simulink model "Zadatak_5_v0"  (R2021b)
settings: Solver=VariableStepAuto  StartTime=0.0  StopTime=0.2  RelTol=1e-3
libraries: ee_lib x5, fl_lib x4, nesl_utility x3, spsSequenceAnalyzerLib x1

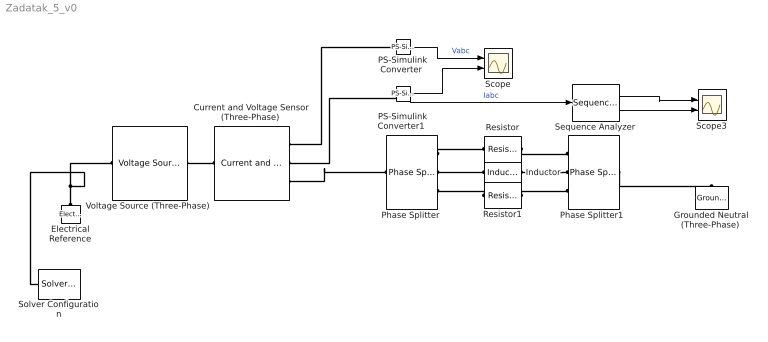
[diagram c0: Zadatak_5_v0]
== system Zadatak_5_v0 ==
  "Current and Voltage Sensor (Three-Phase) " : ee_lib/Sensors & Transducers/Current and Voltage Sensor (Three-Phase)  vMeasurementType=ee.enum.vmeasurement.lg  outputUnit=ee.enum.unit.si  SRated=100e6 V*A  VRated=24e3 V  I_specify=off  I_priority=None  I=[ 0 0 0 ] A  I_nominal_specify=off  I_nominal_unit=A  I_nominal_value=1  V_specify=off  V_priority=None  V=[ 0 0 0 ] V  V_nominal_specify=off  V_nominal_unit=V  V_nominal_value=1
  Electrical Reference : fl_lib/Electrical/Electrical Elements/Electrical Reference
  "Grounded Neutral (Three-Phase) " : ee_lib/Connectors & References/Grounded Neutral (Three-Phase)
  Inductor : fl_lib/Electrical/Electrical Elements/Inductor  l=1 H  r=0 Ohm  g=1e-9 1/Ohm  i_specify=off  i_priority=None  i=0 A  i_nominal_specify=off  i_nominal_unit=A  i_nominal_value=1  v_specify=off  v_priority=None  v=0 V  v_nominal_specify=off  v_nominal_unit=V  v_nominal_value=1  i_L_specify=off  i_L_priority=High  i_L=0 A  i_L_nominal_specify=off  i_L_nominal_unit=A  i_L_nominal_value=1
  "PS-Simulink Converter " : nesl_utility/PS-Simulink Converter  PhysicalDomain=network_engine_domain  SubClassName=ps_output  LeftPortType=input  RightPortType=output  PseudoPeriodic=off  Frequencies=[]  Unit=inherit  AffineConversion=off
  "PS-Simulink Converter1 " : nesl_utility/PS-Simulink Converter  PhysicalDomain=network_engine_domain  SubClassName=ps_output  LeftPortType=input  RightPortType=output  PseudoPeriodic=off  Frequencies=[]  Unit=inherit  AffineConversion=off
  "Phase Splitter " : ee_lib/Connectors & References/Phase Splitter
  "Phase Splitter1 " : ee_lib/Connectors & References/Phase Splitter
  Resistor : fl_lib/Electrical/Electrical Elements/Resistor  R=1000 Ohm  i_specify=off  i_priority=None  i=0 A  i_nominal_specify=off  i_nominal_unit=A  i_nominal_value=1  v_specify=off  v_priority=None  v=0 V  v_nominal_specify=off  v_nominal_unit=V  v_nominal_value=1
  Resistor1 : fl_lib/Electrical/Electrical Elements/Resistor  R=1000 Ohm  i_specify=off  i_priority=None  i=0 A  i_nominal_specify=off  i_nominal_unit=A  i_nominal_value=1  v_specify=off  v_priority=None  v=0 V  v_nominal_specify=off  v_nominal_unit=V  v_nominal_value=1
  Scope : Scope  NumInputPorts=2
  Scope3 : Scope  NumInputPorts=2
  "Sequence Analyzer " : spsSequenceAnalyzerLib/Sequence Analyzer  Freq=50  n=1  seq=Positive Negative Zero  InInit=[1, 0]  Ts=0
  Solver Configuration : nesl_utility/Solver Configuration  PhysicalDomain=network_engine_domain  SubClassName=solver  LeftPortType=input  RightPortType=generic  Tones=[]  Harmonics=[]  SimulateNoise=off  Profile=off  UseLocalSampling=off  EnableSwitchedLinearOptims=on  FrequencyDomain=off  UseCCode=off  RelTol=0.001  AbsTol=1e-06  MinStep=1e-09  ToWorkspace=off  RevertToSquareIcSolve=off  NumHomotopyIterations=100  PhasorMode=off  PhasorModeNumHarmonics=1  DoDC=on  ResidualTolerance=1e-09  UseLocalSolver=off  LocalSolverChoice=NE_BACKWARD_EULER_ADVANCER  LocalSolverSampleTime=0.001  DoFixedCost=off  MaxNonlinIter=3  MaxModeIter=2  ComputeImpulses=off  ImpulseIterations=2  LinearAlgebra=auto  EquationFormulation=NE_TIME_EF  DelaysMemoryBudget=1024  AutomaticFiltering=on  FilteringTimeConstant=0.001  PartitionStorageMethod=AS_NEEDED  PartitionMemoryBudget=1024  PartitionMethod=ROBUST
  "Voltage Source (Three-Phase) " : ee_lib/Sources/Voltage Source (Three-Phase)  vline_rms=380 V  shift=0 deg  freq=50 Hz  impedance_option=0  SShortCircuit=1e6 V*A  XR=15  R=0.01 Ohm  L=3.97e-4 H  harmonic_option=0  harmonic_orders=[5, 7, 11, 13]  harmonic_ratios=[.1, .1, .1, .1]  G_parasitic=0 1/Ohm  I_specify=off  I_priority=None  I=[ 0 0 0 ] A  I_nominal_specify=off  I_nominal_unit=A  I_nominal_value=1
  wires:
  "PS-Simulink Converter "/1 -> Scope/1  "Vabc"
  "PS-Simulink Converter1 "/1 -> Scope/2, "Sequence Analyzer "/1  "Iabc"
  "Sequence Analyzer "/1 -> Scope3/1
  "Sequence Analyzer "/2 -> Scope3/2
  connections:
  Electrical Reference/LConn1 -- Solver Configuration/RConn1 -- "Voltage Source (Three-Phase) "/LConn1
  "Phase Splitter1 "/LConn1 -- "Grounded Neutral (Three-Phase) "/LConn1
  "Phase Splitter "/RConn1 -- Resistor/LConn1
  Resistor/RConn1 -- "Phase Splitter1 "/RConn1
  "Voltage Source (Three-Phase) "/RConn1 -- "Current and Voltage Sensor (Three-Phase) "/LConn1
  "Current and Voltage Sensor (Three-Phase) "/RConn3 -- "Phase Splitter "/LConn1
  "PS-Simulink Converter "/LConn1 -- "Current and Voltage Sensor (Three-Phase) "/RConn1
  "PS-Simulink Converter1 "/LConn1 -- "Current and Voltage Sensor (Three-Phase) "/RConn2
  Resistor1/LConn1 -- "Phase Splitter "/RConn3
  Resistor1/RConn1 -- "Phase Splitter1 "/RConn3
  "Phase Splitter "/RConn2 -- Inductor/LConn1
  Inductor/RConn1 -- "Phase Splitter1 "/RConn2
